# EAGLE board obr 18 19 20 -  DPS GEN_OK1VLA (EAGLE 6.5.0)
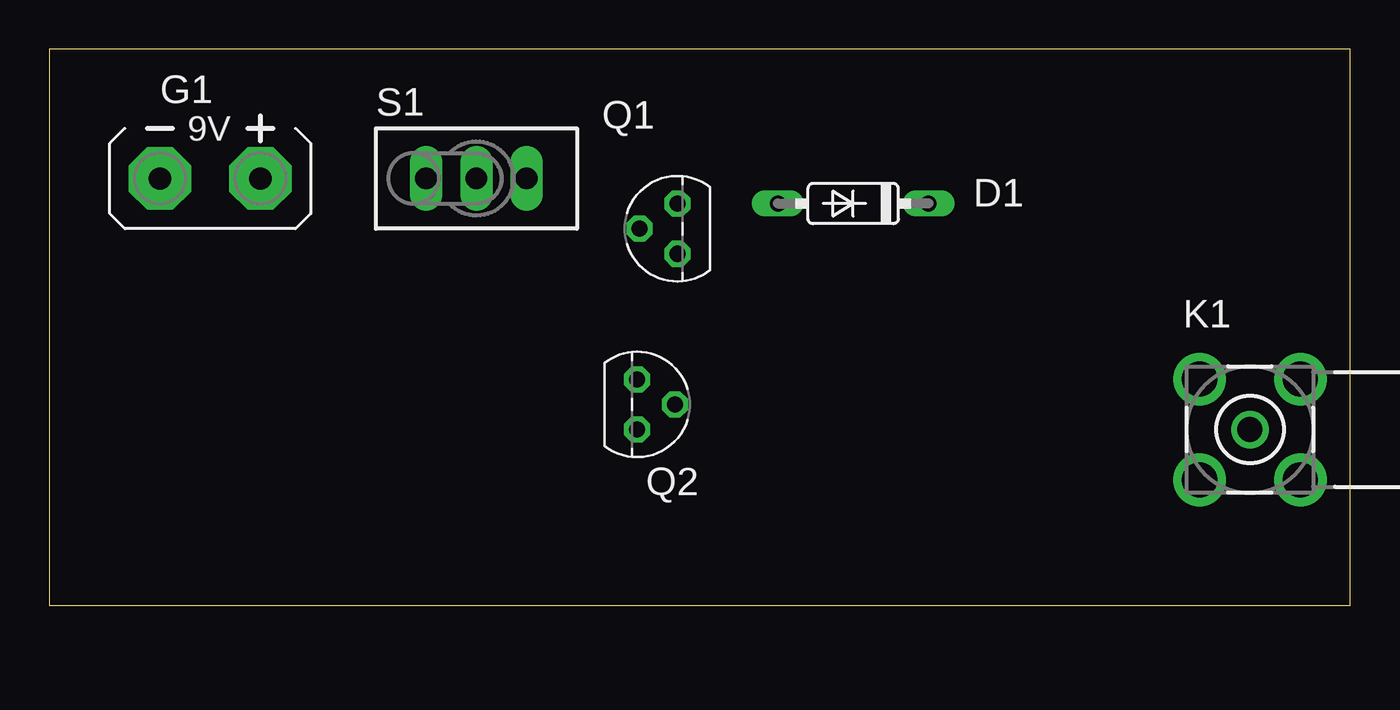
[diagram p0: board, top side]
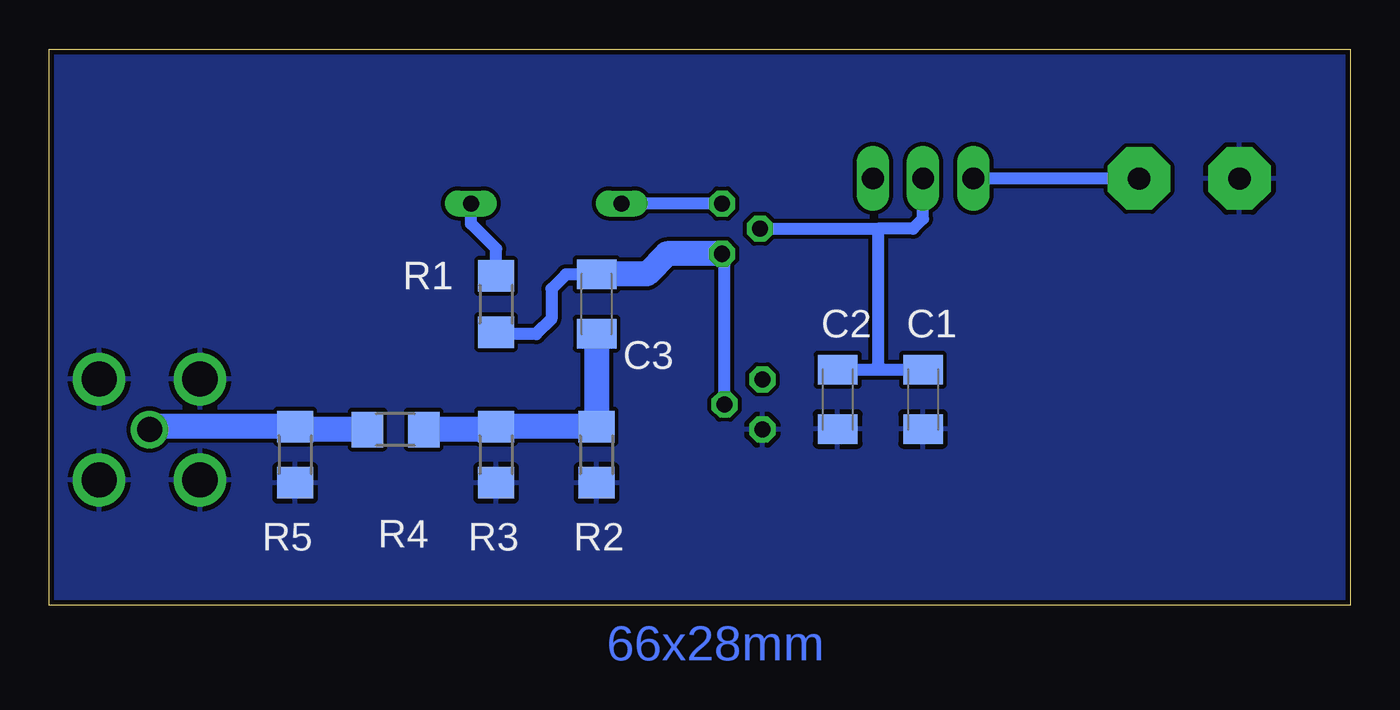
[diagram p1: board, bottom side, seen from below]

Size 65.77 x 28.12 mm. Coordinates in mm from the lower left corner, seen from the top.
Outline: 0,0 65.77,0 65.77,28.12 0,28.12 0,0
Copper layers (1*16): Top 0.035mm / dielectric 1.5mm / Bottom 0.035mm
Design rules "default *": minimum track width 10mil, minimum drill 24mil, track to track 8mil, track to pad 8mil, pad to pad 8mil, via to via 8mil, smd to smd 8mil, copper to edge 10mil, drill to drill 8mil, minimum pad ring 10mil, minimum via ring 8mil, stop-mask expansion 4mil, vias tented up to drill 0mil, thermal gap 10mil

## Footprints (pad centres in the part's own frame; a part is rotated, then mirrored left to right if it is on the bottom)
C1206K = smd 1.5 x 2: 1 -1.5,0; 2 1.5,0
DO35-7 = drill 0.813 long: A 3.81,0; C -3.81,0
AB9V = drill 1.118 pad 3.15 octagon: + 0,2.54; - 0,-2.54
BU-SMA-H = drill 1.27: 1 0,0 | drill 1.778: 2 -2.55,2.55; 3 2.55,2.55; 4 2.55,-2.55; 5 -2.55,-2.55
TO92 = drill 0.813 octagon: 1 1.27,0; 2 0,1.905; 3 -1.27,0
R1206 = smd 1.6 x 1.803: 1 -1.422,0; 2 1.422,0
TL3XPO = drill 1.1 pad 1.422 long: 1 -2.54,0; 2 0,0; 3 2.54,0

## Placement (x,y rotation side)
C1  100nF  [C1206K]  21.59,10.41 270 bottom
C2  1nF  [C1206K]  25.91,10.41 270 bottom
C3  1nF  [C1206K]  38.1,15.24 90 bottom
D1  1N4148  [DO35-7]  40.64,20.32 180 top
G1  AB9V  [AB9V]  8.13,21.59 270 top
K1  [BU-SMA-H]  60.71,8.89 0 top
Q1  BF245  [TO92]  31.75,19.05 90 top
Q2  BF199  [TO92]  29.72,10.16 270 top
R1  2K2  [R1206]  43.18,15.24 90 bottom
R2  50R  [R1206]  38.1,7.62 90 bottom
R3  294  [R1206]  43.18,7.62 90 bottom
R4  17,5  [R1206]  48.26,8.89 0 bottom
R5  294  [R1206]  53.34,7.62 90 bottom
S1  TL32PO  [TL3XPO]  21.59,21.59 0 top

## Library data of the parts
C1-C3 = rcl
D1 = diode
G1 = battery
K1 = con-coax; OC_FARNELL: unknown; OC_NEWARK: unknown
Q1 = transistor-fet
Q2 = transistor-npn
R1-R5 = resistor
S1 = switch

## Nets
GND: C1.2 C2.2 G1.- K1.2 K1.3 K1.4 K1.5 Q2.1 R2.1 R3.1 R5.1
N$1: C1.1 C2.1 Q1.2 S1.2
N$2: D1.A Q1.1
N$3: C3.2 Q1.3 Q2.2 R1.1
N$4: D1.C R1.2
N$5: C3.1 R2.2 R3.2 R4.2
N$6: K1.1 R4.1 R5.2
N$7: G1.+ S1.1

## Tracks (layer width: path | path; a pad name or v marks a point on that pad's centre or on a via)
GND
  pour Bottom: 0.25,27.94 65.53,27.94 65.53,0.25 0.25,0.25
  pour Bottom (isolate 0.406): 0.25,27.94 65.53,27.94 65.53,0.25 0.25,0.25
N$1
  Bottom 0.61: Q1.2 23.88,19.05 | S1.2 21.59,19.56 22.1,19.05 23.88,19.05 | C1.1 23.62,11.91 | 23.62,11.91 C2.1 | 23.88,19.05 23.88,12.17 23.62,11.91
N$2
  Bottom 0.61: Q1.1 D1.A
N$3
  Bottom 0.61: C3.2 39.65,16.74 40.39,16 40.39,14.48 41.15,13.72 43.08,13.72 R1.1 | Q2.2 31.62,17.65 Q1.3
  Bottom 1.27: Q1.3 34.54,17.78 35.56,16.76 38.08,16.76 C3.2
N$4
  Bottom 0.61: R1.2 43.18,18.03 44.45,19.3 D1.C
N$5
  Bottom 0.61: 43.18,8.89 R3.2
  Bottom 1.27: C3.1 R2.2 R3.2 | 43.18,8.89 R4.2
N$6
  Bottom 0.61: 53.34,8.89 R5.2
  Bottom 1.27: R4.1 53.19,8.89 R5.2 60.55,9.04 K1.1
N$7
  Bottom 0.61: G1.+ S1.1

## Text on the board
Bottom: 66x28mm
